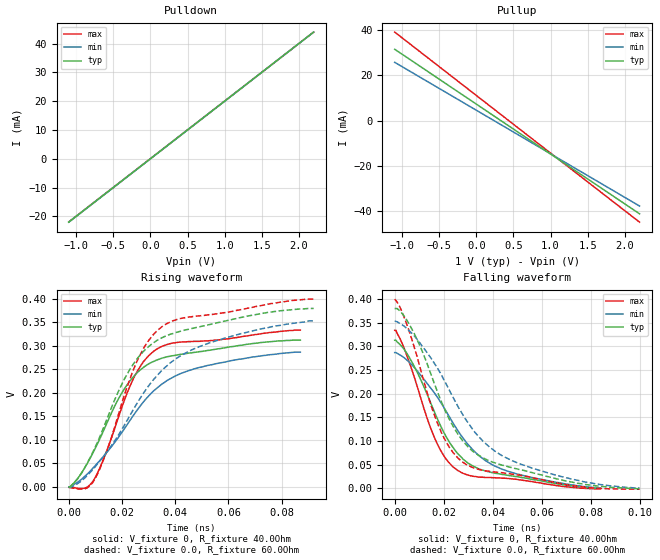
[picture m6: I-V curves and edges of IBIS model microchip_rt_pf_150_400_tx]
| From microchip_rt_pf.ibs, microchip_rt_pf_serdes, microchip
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[Model]   microchip_rt_pf_150_400_tx
Model_type   Output
Polarity   Non-Inverting
Enable   Active-High
Vmeas = 0.5
|   typ   min   max
C_comp   0.407p  0.407p  0.407p
[Voltage Range]   1.0  0.9  1.1
[Temperature Range]   27  27  27
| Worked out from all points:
|   slope of the pulldown table from 0 to 0.15 V, typ, clamps not added: 50 ohm
|   slope of the pullup table from 0 to 0.15 V, typ, clamps not added: 45.4 ohm
|   rising waveform, V_fixture 0, R_fixture 40.0Ohm: 20-80 % time 18.9ps typ, 26ps min, 14.6ps max; typ from 0 V to 0.312 V
|   rising waveform, V_fixture 0.0, R_fixture 60.0Ohm: 20-80 % time 22ps typ, 29.3ps min, 16.7ps max; typ from 0 V to 0.38 V
|   falling waveform, V_fixture 0, R_fixture 40.0Ohm: 20-80 % time 19.1ps typ, 25.2ps min, 14.6ps max; typ from 0.312 V to 0 V
|   falling waveform, V_fixture 0.0, R_fixture 60.0Ohm: 20-80 % time 22.6ps typ, 29.4ps min, 16.7ps max; typ from 0.38 V to -0.001 V
[Pullup]
|   X   TYP   MIN   MAX
-1.1V     31.57mA    25.8mA     39.15mA
1.01V     -14.91mA   -14.79mA   -14.54mA
1.089V    -16.64mA   -16.31mA   -16.54mA
2.2V      -41.12mA   -37.68mA   -44.81mA
[Pulldown]
|   X   TYP   MIN   MAX
-1.1V     -21.97mA   -22.01mA   -21.92mA
1.033V    20.66mA    20.65mA    20.68mA
1.089V    21.79mA    21.77mA    21.8mA
2.2V      44mA       44mA       44mA
[Ramp]
R_load = 50.0Ohm
|   typ   min   max
dV/dt_r   1.88E-1V/1.89E-2ns   1.72E-1V/2.60E-2ns   2.01E-1V/1.46E-2ns
dV/dt_f   1.88E-1V/1.91E-2ns   1.72E-1V/2.52E-2ns   2.01E-1V/1.46E-2ns
[Rising Waveform]
V_fixture   = 0
V_fixture_min = 0
V_fixture_max = 0
R_fixture   = 40.0Ohm
|   Time   V(typ)   V(min)   V(max)
0s        -500uV     0V         -1mV
6ps       40.7mV     22.19mV    -3.005mV
9ps       71.27mV    39.24mV    10.94mV
13ps      118.7mV    64.58mV    58.36mV
18ps      180.1mV    100.1mV    136.9mV
24ps      232.4mV    149.7mV    226.9mV
28ps      253.8mV    180.3mV    265.9mV
33ps      269.7mV    209.4mV    293mV
49ps      287.5mV    253.9mV    309.5mV
87ps      312mV      286.5mV    333.5mV
[Rising Waveform]
V_fixture   = 0.0
V_fixture_min = 0.0
V_fixture_max = 0.0
R_fixture   = 60.0Ohm
|   Time   V(typ)   V(min)   V(max)
0s        -500uV     -500uV     -1.5mV
6ps       40.72mV    18.77mV    -4.524mV
10ps      85.08mV    43.29mV    18.53mV
14ps      139.4mV    72mV       71.96mV
19ps      207.4mV    113.2mV    160.5mV
25ps      267.2mV    171.5mV    259mV
30ps      298.3mV    214.8mV    311.4mV
35ps      317.2mV    248mV      340.6mV
53ps      345.3mV    306.5mV    366.3mV
92ps      379.5mV    353mV      399.5mV
[Falling Waveform]
V_fixture   = 0
V_fixture_min = 0
V_fixture_max = 0
R_fixture   = 40.0Ohm
|   Time   V(typ)   V(min)   V(max)
0s        312.5mV    286.5mV    333.5mV
3ps       298.8mV    278.8mV    306.4mV
7ps       266.9mV    260.7mV    250.5mV
13ps      201.6mV    223mV      151.5mV
17ps      151.8mV    195.5mV    97.86mV
21ps      108.9mV    162.5mV    61.54mV
25ps      77.82mV    128.1mV    40.35mV
33ps      44.24mV    75.54mV    24.7mV
43ps      30mV       41.9mV     21.67mV
84ps      -497.5uV   500uV      -1.5mV
[Falling Waveform]
V_fixture   = 0.0
V_fixture_min = 0.0
V_fixture_max = 0.0
R_fixture   = 60.0Ohm
|   Time   V(typ)   V(min)   V(max)
0s        379.5mV    353mV      399.5mV
3ps       369.4mV    345.3mV    372.5mV
8ps       326.6mV    321.8mV    297.7mV
14ps      252.1mV    280.7mV    188.9mV
19ps      183.7mV    240.2mV    118.2mV
28ps      98.53mV    153.7mV    54.32mV
36ps      64.32mV    99.58mV    37.71mV
48ps      43.38mV    57.99mV    29.67mV
77ps      8.701mV    13.86mV    2.528mV
100ps     -995uV     500uV      -2mV
[Algorithmic Model]
Executable Linux_gcc5.4_64   MPF300T-TX_LX64.so   MPF300T-TX-R150_400.ami
Executable Windows_cl18.00.40629_64 MPF300T-TX_WIN64.dll  MPF300T-TX-R150_400.ami
Executable Windows_cl18.00.40629_32 MPF300T-TX_WIN32.dll  MPF300T-TX-R150_400.ami
[End Algorithmic Model]
